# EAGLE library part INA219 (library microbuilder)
INA219 - I2C Current/Power Monitor Voltage Range: 0-26V Accuracy: 0.5% Temperature: -40°C - 125°C
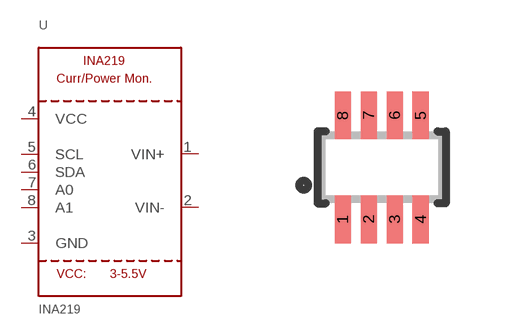
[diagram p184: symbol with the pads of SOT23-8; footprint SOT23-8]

Designator prefix U

## INA219  [SOT23-8]
1  VIN+
2  VIN-
3  GND
4  VCC
5  SCL
6  SDA
7  A0
8  A1

## Footprint SOT23-8 (pad centres in mm)
Source: http://www.ti.com/lit/ml/mpds099c/mpds099c.pdf
smd 0.4 x 1.2: 1 -0.975,-1.3; 2 -0.325,-1.3; 3 0.325,-1.3; 4 0.975,-1.3; 5 0.975,1.3; 6 0.325,1.3; 7 -0.325,1.3; 8 -0.975,1.3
